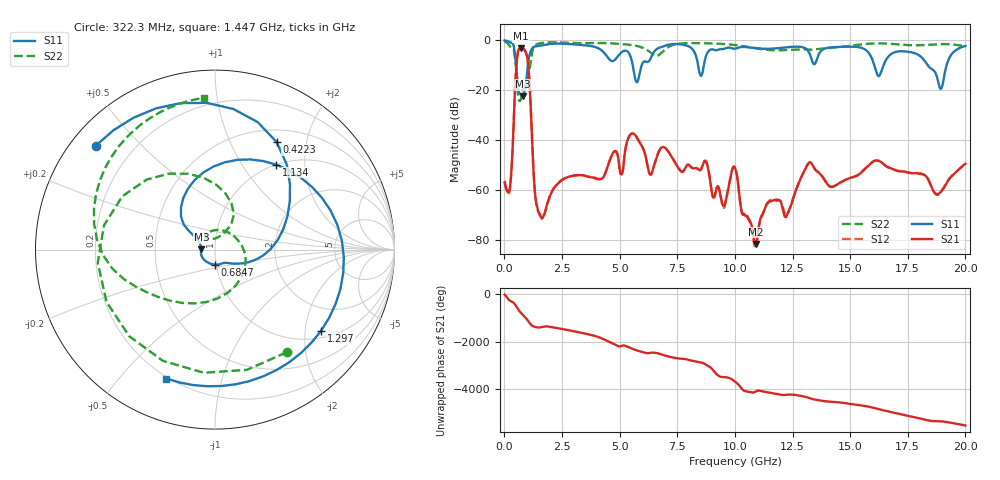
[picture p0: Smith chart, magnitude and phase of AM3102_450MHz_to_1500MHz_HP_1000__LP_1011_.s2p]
!Agilent Technologies,E8364B,MY43040894,A.07.50.67
!Agilent E8364B: A.07.50.67
!Date: Thursday, January 11, 2018 05:59:10
!Correction: S11(Full 2 Port(1,2))
!S21(Full 2 Port(1,2))
!S12(Full 2 Port(1,2))
!S22(Full 2 Port(1,2))
!S2P File: Measurements: S11, S21, S12, S22:
# Hz S  dB  R 50
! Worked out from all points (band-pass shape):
!   1601 points, 10 MHz to 20 GHz, reference 50 ohm
!   highest |S21| = -3.14 dB at 722.1 MHz (marker M1); lowest = -81.7 dB at 10.92 GHz (marker M2)
!   |S21| within 3 dB of the highest: 563.4 MHz to 975.3 MHz (412 MHz wide, 53.5 % of centre)
!   lowest |S11| = -22.4 dB at 797.1 MHz (marker M3), VSWR 1.16, Z = 43 + j0.185 ohm
!   |S11| at or under -10 dB: 507.8 MHz to 1.015 GHz (507.2 MHz wide, 66.6 % of centre); 5.569 GHz to 5.957 GHz (387.5 MHz wide, 6.72 % of centre); 18.37 GHz to 19.18 GHz (818.6 MHz wide, 4.36 % of centre)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
!   |S22| runs from -24.3 to -0.5 dB; largest |S21 - S12| = 0.001
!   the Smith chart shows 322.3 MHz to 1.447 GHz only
!   S11 on the Smith chart (normalised r, x): 322.3 MHz: 0.07, +0.37; 422.3 MHz: 0.66, +1.52; 684.7 MHz: 0.98, -0.16; 1.134 GHz: 1.00, +1.44; 1.297 GHz: 1.20, -2.43; 1.447 GHz: 0.19, -0.67
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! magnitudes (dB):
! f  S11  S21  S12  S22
! 10 MHz  -0.1  -57.1  -56.3  -0.5
! 322.3 MHz  -1.1  -49.6  -50.2  -3.1
! 422.3 MHz  -3.2  -28.2  -28.1  -4.5
! 684.7 MHz  -21.6  -3.2  -3.2  -24.2
! 722.1 MHz  -21.7  -3.1  -3.1  -23.4
! 797.1 MHz  -22.4  -3.3  -3.3  -19.8
! 1.134 GHz  -4.7  -25.0  -25.0  -9.1
! 1.297 GHz  -2.6  -57.4  -57.6  -2.4
! 1.447 GHz  -2.3  -67.8  -68.1  -1.4
! 3.346 GHz  -1.9  -54.0  -54.2  -1.1
! 5.082 GHz  -4.8  -53.8  -53.7  -1.5
! 5.745 GHz  -16.8  -39.0  -39.0  -2.3
! 6.332 GHz  -7.5  -53.9  -53.9  -4.8
! 6.682 GHz  -3.1  -45.0  -45.0  -6.0
! 8.731 GHz  -6.8  -48.4  -48.4  -1.2
! 9.505 GHz  -3.5  -66.5  -67.1  -1.5
! 10.01 GHz  -3.4  -51.2  -51.1  -1.9
! 10.92 GHz  -3.2  -81.7  -82.1  -3.2
! 13.34 GHz  -8.0  -49.6  -49.6  -3.7
! 16.68 GHz  -6.4  -51.0  -51.1  -1.3
! 18.93 GHz  -19.4  -60.9  -61.0  -1.5
! 20 GHz  -2.3  -49.5  -49.4  -2.3
